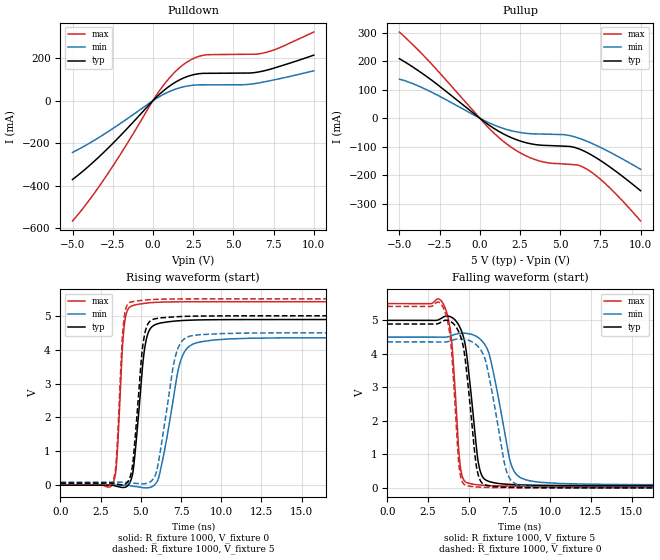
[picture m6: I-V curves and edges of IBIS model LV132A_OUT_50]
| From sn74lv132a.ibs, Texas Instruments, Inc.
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[Model]   LV132A_OUT_50
Model_type  Output
Vref =   0
Rref =   1000
Cref =   50p
Vmeas =   2.5
| variable   typ   min   max
C_comp   7.51pF   3.36pF   18.13pF
| C_pullup   5.47pF   3.36pF   7.06pF
| C_pulldown   9.55pF   4.02pF   18.13pF
[Temperature Range]   40   100   -40
| Ambient temperature   25   85   -40
[Voltage range]   5   4.5   5.5
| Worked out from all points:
|   slope of the pulldown table from 0 to 0.75 V, typ, clamps not added: 14.3 ohm
|   slope of the pullup table from 0 to 0.75 V, typ, clamps not added: 24.2 ohm
|   rising waveform, R_fixture 1000, V_fixture 0: 20-80 % time 553ps typ, 957ps min, 345ps max; typ from 0 V to 4.89 V
|   falling waveform, R_fixture 1000, V_fixture 5: 20-80 % time 644ps typ, 1.03ns min, 440ps max; typ from 5 V to 0.063 V
|   rising waveform, R_fixture 1000, V_fixture 5: 20-80 % time 513ps typ, 862ps min, 333ps max; typ from 0.063 V to 5 V
|   falling waveform, R_fixture 1000, V_fixture 0: 20-80 % time 621ps typ, 960ps min, 432ps max; typ from 4.89 V to 0 V
[Pulldown]
| LV132A_OUT_50
|   Voltage   I(typ)   I(min)   I(max)
-5V       -370.5mA   -243.2mA   -565.6mA
-3.94V    -304.5mA   -199.5mA   -465.4mA
-2.795V   -223.4mA   -145.9mA   -342.3mA
435mV     32.11mA    20.49mA    49.82mA
1.13V     73.88mA    46.39mA    116mA
1.825V    103.9mA    63.85mA    165.5mA
2.515V    122.1mA    72.81mA    198.2mA
3.205V    128.6mA    74.3mA     214.5mA
5.71V     129.9mA    75.47mA    218.1mA
6.99V     141.9mA    89.41mA    226.2mA
7.965V    163.5mA    104.8mA    251.8mA
10V       214.2mA    140.6mA    322.8mA
[Pullup]
| LV132A_OUT_50
|   Voltage   I(typ)   I(min)   I(max)
-5V       209.3mA    137.2mA    303.1mA
-3.125V   139.2mA    95.22mA    198.4mA
450mV     -19.36mA   -13.01mA   -28.02mA
1.57V     -58.06mA   -37.82mA   -86.01mA
2.55V     -80.84mA   -50.67mA   -123mA
3.53V     -93.27mA   -55.26mA   -147.2mA
4.35V     -96.18mA   -56.39mA   -157.6mA
5.655V    -99.78mA   -61.94mA   -162.6mA
6.11V     -106.6mA   -69.34mA   -164.9mA
6.61V     -119.1mA   -79.89mA   -177.6mA
8.015V    -168.6mA   -117.3mA   -241.3mA
10V       -255.1mA   -179.6mA   -361.5mA
[Ramp]
| LV132A_OUT_50
| variable   typ   min   max
dV/dt_r   2.97/5.64E-10   2.66/9.76E-10   3.28/3.57E-10
dV/dt_f   3.04/6.69E-10   2.72/1.06E-09   3.36/4.68E-10
R_load = 1000
[Rising Waveform]
| LV132A_OUT_50
R_fixture =   1000
C_fixture =   0
L_fixture =   0
V_fixture =   0
V_fixture_min = 0
V_fixture_max = 0
|   Time   V(typ)   V(min)   V(max)
0s        1.811nV    6.144nV    1.238nV
3.275ns   -4.836mV   114.1uV    58.81mV
3.51ns    -33.33mV   506.8uV    780.2mV
3.99ns    -62.78mV   2.125mV    4.788V
4.71ns    1.284V     -40.2mV    5.328V
5.535ns   4.579V     -70.44mV   5.384V
6.165ns   4.781V     324.4mV    5.402V
7.51ns    4.859V     3.719V     5.413V
8.69ns    4.879V     4.228V     5.415V
50ns      4.89V      4.354V     5.415V
[Falling Waveform]
| LV132A_OUT_50
R_fixture =   1000
C_fixture =   0
L_fixture =   0
V_fixture =   5
V_fixture_min = 4.5
V_fixture_max = 5.5
|   Time   V(typ)   V(min)   V(max)
0s        5V         4.5V       5.5V
3.485ns   5.11V      4.496V     5.447V
3.945ns   5.091V     4.541V     4.423V
4.5ns     4.746V     4.61V      575.5mV
5.145ns   2.799V     4.586V     120.2mV
5.55ns    880.1mV    4.498V     89.98mV
5.87ns    313.9mV    4.353V     77.25mV
7.61ns    99.89mV    692.8mV    52.55mV
8.75ns    81.27mV    211.5mV    48.32mV
50ns      63.04mV    88.01mV    45mV
[Rising Waveform]
| LV132A_OUT_50
R_fixture =   1000
C_fixture =   0
L_fixture =   0
V_fixture =   5
V_fixture_min = 4.5
V_fixture_max = 5.5
|   Time   V(typ)   V(min)   V(max)
0s        63.04mV    88.01mV    45mV
3.26ns    59.48mV    88.13mV    119.3mV
3.485ns   34.87mV    88.47mV    819mV
3.915ns   15.81mV    90.23mV    4.739V
4.405ns   363.2mV    70.54mV    5.409V
5.17ns    4.275V     41.31mV    5.459V
5.935ns   4.917V     334.7mV    5.486V
7.16ns    4.971V     3.818V     5.497V
8.2ns     4.989V     4.416V     5.499V
50ns      5V         4.5V       5.5V
[Falling Waveform]
| LV132A_OUT_50
R_fixture =   1000
C_fixture =   0
L_fixture =   0
V_fixture =   0
V_fixture_min = 0
V_fixture_max = 0
|   Time   V(typ)   V(min)   V(max)
0s        4.891V     4.356V     5.416V
3.465ns   4.99V      4.352V     5.348V
3.895ns   4.962V     4.388V     4.359V
4.42ns    4.621V     4.446V     593.7mV
4.9ns     3.333V     4.417V     60.81mV
5.435ns   763.2mV    4.284V     28.28mV
5.695ns   232.6mV    4.146V     20.79mV
7.295ns   19.17mV    536.6mV    4.763mV
8.205ns   9.798mV    73.56mV    2.368mV
50ns      64.2nV     411.6nV    3.009nV
